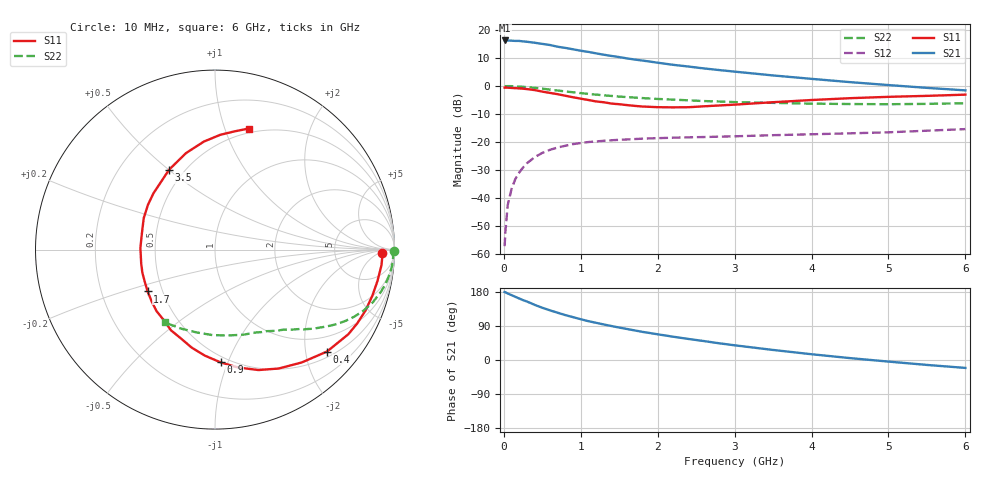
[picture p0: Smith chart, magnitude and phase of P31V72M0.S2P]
! SIEMENS Small Signal Semiconductors
! BFP181
! Si NPN RF Bipolar Junction Transistor in SOT143
! VCE = 1.75 V  IC = 2 mA
! Common Emitter S-Parameters:  March  1996
# GHz  S  MA  R  50
!  f  S11  S21  S12  S22
! GHz  MAG  ANG  MAG  ANG  MAG  ANG  MAG  ANG
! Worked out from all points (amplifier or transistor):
!   36 points, 10 MHz to 6 GHz, reference 50 ohm
!   highest |S21| = 16.2 dB at 10 MHz (marker M1)
!   |S21| within 3 dB of that: start of sweep to 869.7 MHz
!   unconditionally stable (mu >= 1): 2.381 GHz to end of sweep
!   at 250 MHz: K = 0.12, MSG = 22.5 dB, |S12| = -29.0 dB
!   at 1.4 GHz: K = 0.66, MSG = 15.0 dB, |S12| = -19.3 dB
!   at 6 GHz: K = 1.16, MAG = 4.5 dB, |S12| = -15.4 dB
!   S11 on the Smith chart (normalised r, x): 10 MHz: 25, -8; 400 MHz: 0.62, -2.45; 900 MHz: 0.45, -0.94; 1.7 GHz: 0.41, -0.24; 3.5 GHz: 0.41, +0.50; 6 GHz: 0.46, +1.21
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0.01  0.9307 -1.3  6.463 179.3  0.0014 87.8  0.9974 -0.4
0.02  0.9332 -2.1  6.455 178.8  0.0025 83.7  0.9902 -0.9
0.05  0.9316 -5.4  6.453 175.6  0.0075 87.8  0.9935 -2.5
0.1  0.9219 -11.0  6.403 171.2  0.0146 82.5  0.9909 -5.0
0.2  0.9051 -21.9  6.336 162.3  0.0287 77.0  0.9754 -9.8
0.3  0.8799 -32.4  6.125 154.4  0.0419 70.6  0.953 -14.4
0.4  0.8439 -42.3  5.889 145.6  0.0538 65.0  0.9269 -18.5
0.5  0.7928 -52.5  5.617 137.8  0.0642 59.0  0.8951 -22.3
0.6  0.7517 -61.8  5.36 131.0  0.0729 54.4  0.8615 -25.7
0.7  0.7137 -70.1  4.997 124.7  0.0802 50.5  0.829 -28.6
0.8  0.669 -79.0  4.761 118.5  0.086 46.6  0.7994 -31.1
0.9  0.6289 -87.2  4.497 113.0  0.0921 43.1  0.7714 -33.3
1.1  0.5616 -103.3  4.04 102.4  0.1003 37.5  0.7214 -37.2
1.4  0.4852 -126.2  3.422 89.6  0.1079 31.0  0.6634 -42.1
1.7  0.4419 -148.2  2.956 78.1  0.1133 26.6  0.6205 -45.9
1.9  0.4247 -162.3  2.717 71.1  0.1164 24.3  0.597 -48.3
2.2  0.4158 178.6  2.381 61.5  0.1198 21.8  0.5706 -52.2
2.8  0.4491 146.3  1.919 44.1  0.125 18.2  0.5282 -60.5
3.5  0.5134 119.9  1.539 26.5  0.1328 15.4  0.4997 -71.6
4.5  0.6054 95.8  1.17 5.0  0.1433 12.2  0.4765 -91.7
5.5  0.6663 80.9  0.925 -13.0  0.1596 10.8  0.4795 -113.4
6  0.7 74.5  0.834 -20.9  0.1704 8.7  0.4928 -124.7
